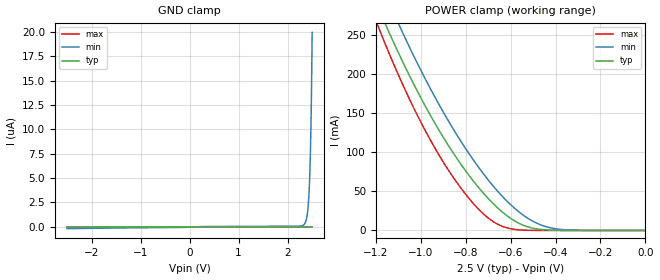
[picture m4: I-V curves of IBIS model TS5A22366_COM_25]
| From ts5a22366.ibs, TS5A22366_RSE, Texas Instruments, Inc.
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[Model]   TS5A22366_COM_25
Model_type  Terminator
| variable   typ   min   max
C_comp   101.99pF   71.02pF   125.05pF
| C_tri-state   101.99pF   71.02pF   125.05pF
[Temperature Range]   40   100   -40
| Ambient temperature   25   85   -40
[Voltage range]   2.5   2.3   2.7
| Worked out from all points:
|   POWER clamp passes 1 mA (typ) near -0.45 V on its own axis
[GND Clamp]
| TS5A22366_COM_25
|   Voltage   I(typ)   I(min)   I(max)
-2.5V     -4.818nA   -192.8nA   -2.936nA
2.325V    2.805nA    185.4nA    2.348nA
2.365V    2.856nA    481.7nA    2.391nA
2.395V    2.897nA    1.091uA    2.423nA
2.42V     2.939nA    2.201uA    2.45nA
2.44V     2.984nA    3.862uA    2.471nA
2.45V     3.015nA    5.105uA    2.482nA
2.46V     3.054nA    6.738uA    2.493nA
2.475V    3.139nA    10.18uA    2.509nA
2.485V    3.223nA    13.35uA    2.519nA
2.49V     3.277nA    15.28uA    2.525nA
2.5V      3.417nA    19.97uA    2.536nA
[POWER Clamp]
| TS5A22366_COM_25
|   Voltage   I(typ)   I(min)   I(max)
-2.5V     1.643A     1.675A     1.79A
-1.19V    285.9mA    325mA      261.7mA
-1.175V   275.8mA    314.7mA    250.9mA
-1.14V    253mA      291.3mA    226.3mA
-1.08V    215.8mA    253mA      186.7mA
-925mV    131.4mA    164.6mA    99.64mA
-800mV    76.23mA    104.8mA    46.32mA
-690mV    38.03mA    61.25mA    13.8mA
-570mV    10.25mA    25.39mA    996.9uA
-490mV    2.318mA    10.17mA    78.92uA
-395mV    223.8uA    1.991mA    2.198uA
0V        0A         0A         0A
